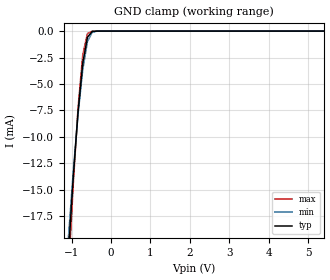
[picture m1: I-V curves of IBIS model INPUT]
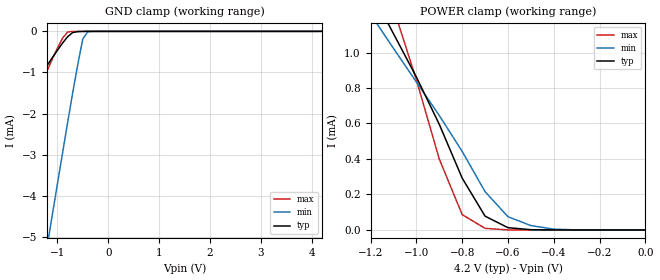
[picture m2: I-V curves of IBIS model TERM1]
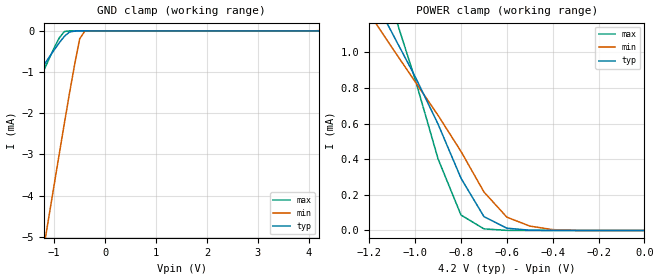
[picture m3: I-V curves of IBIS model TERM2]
|   PERICOM SEMICONDUCTOR CORP
|   IBIS Model of PI3A223
|   Product Family: 3A
|   UQFN-10 (ZM) Package
[IBIS Ver] 3.2
[Comment char] |_char
[File Name] pi3a223_zm_42v.ibs
[File Rev] 1.0
[Source] File originated at Pericom Semiconductor Corp.
[Date] 08/04/17
[Disclaimer] (C) Copyright PERICOM Semiconductor Corporation
   All rights reserved
  Pericom Semiconductor Corporation hereby grants the user of
  this IBIS model a non-exclusive, nontransferable license to
  use this IBIS model under the following terms.
  This IBIS model is provided on an "AS IS" basis and Pericom
  makes absolutely no warranty with respect to the information
  contained herein. PERICOM DISCLAIMS AND CUSTOMER WAIVES ALL
  WARRANTIES, EXPRESSED OR IMPLIED, INCLUDING WARRANTIES OF
  MERCHANTABILITY OR FITNESS FOR A PARTICULAR PURPOSE. The
  entire risk as to quality and performance is with the customer.
  Accordingly, in no event shall the company be liable for any
  damages, whether in contract or tort, including any lost
  profits or other incidental, consequential, exemplary, or
  punitive damages arising out of the use or application of the
  IBIS model provided in this package. Further, Pericom reserves
  the right to make changes without notice to any product herein
  to improve reliability, function, or design. Pericom does not
  convey any license under patent rights or any other intellectual
  property rights, including those of third parties.
  The user is granted this license only to use the IBIS model
  and is not granted rights to sell, load, rent, lease or license
  the IBIS model in whole or in part, or in modified form to anyone
  other than user. User may modify the IBIS model to suit its specific
  application but rights to derivative works and such modifications
  shall belong to Pericom.
  Pericom is not obligated to provide maintenance or support
  for the licensed IBIS model.
  Contact Pericom at ATTN: APPLICATION ENGINEERING / IBIS MODELS
  2380 Bering Drive, San Jose, CA 95131
[Component] PI3A223
[Manufacturer] Pericom Semiconductor Corp.
[Package]
| variable   typ   min   max
R_pkg   0.10120ohm   0.09060ohm   0.11180ohm
L_pkg   1.24800nH   1.01600nH   1.48000nH
C_pkg   0.22300pF   0.20300pF   0.24400pF
[Pin] signal_name   model_name   R_pin   L_pin   C_pin
1   VDD   POWER   0.10120   1.24800nH   0.22300pF
2   NO1   TERM1   0.10120   1.24800nH   0.22300pF
3   COM1   TERM2   0.11180   1.48000nH   0.24400pF
4   IN1   INPUT   0.09060   1.01600nH   0.20200pF
5   NC1   TERM1   0.11180   1.48000nH   0.24400pF
6   GND   GND   0.10120   1.24800nH   0.22300pF
7   NC2   TERM1   0.10120   1.24800nH   0.22300pF
8   IN2   INPUT   0.11180   1.48000nH   0.24400pF
9   COM2   TERM2   0.09060   1.01600nH   0.20200pF
10   NO2   TERM1   0.11180   1.48000nH   0.24400pF
[Series Switch Groups]
On 1 /
Off 2 /
[Series Pin Mapping]   pin_2   model_name  function_table_group
5   3   SWITCH1   1
2   3   SWITCH1   2
7   9   SWITCH1   1
10   9   SWITCH1   2
|   Model SWITCH1
[Model] SWITCH1
Model_type Series_switch
| variable   typ   min   max
C_comp   67.00pF   66.50pF   67.50pF
[Voltage Range]   4.2000V   3.7800V   4.6200V
[GND Clamp Reference]   0.0000V   0.0000V   0.0000V
[POWER Clamp Reference]   4.2000V   3.7800V   4.6200V
[Temperature Range]   25   85   -40
[On]
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[OFF]
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| Models and submodels in the file (4): INPUT (Input), SWITCH1 (Series_switch), TERM1 (Terminator), TERM2 (Terminator)
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|   Model INPUT
[Model] INPUT
Model_type Input
Vinl = 420mV
Vinh = 2.94V
| variable   typ   min   max
C_comp   0.950pF   0.940pF   0.960pF
[Voltage Range]   4.2000V   3.7800V   4.6200V
[GND Clamp Reference]   0.0000V   0.0000V   0.0000V
[POWER Clamp Reference]   4.2000V   3.7800V   4.6200V
[Temperature Range]   25   85   -40
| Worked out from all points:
|   GND clamp passes 1 mA (typ) near -0.62 V on its own axis
[GND Clamp]
| Voltage   I(typ)   I(min)   I(max)
-4.2V     -233.5mA   -213.1mA   -261.7mA
-1.08V    -20.87mA   -19.38mA   -22.91mA
-960mV    -13.8mA    -13.29mA   -14.48mA
-840mV    -7.703mA   -7.939mA   -7.326mA
-720mV    -3.053mA   -3.654mA   -2.254mA
-600mV    -576.6uA   -991.2uA   -224.1uA
-480mV    -38.17uA   -117.3uA   -5.86uA
-240mV    -22.46nA   -288.9nA   -320.8pA
8.4V      1.541nA    46.91nA    172.2pA
[POWER Clamp]   |Note: Vtable = Vcc - Voutput
| Voltage   I(typ)   I(min)   I(max)
-4.2V     0A         0A         0A
0V        0A         0A         0A
|   Model TERM1
[Model] TERM1
Model_type Terminator
| variable   typ   min   max
C_comp   26.00pF   25.80pF   26.20pF
[Voltage Range]   4.2000V   3.7800V   4.6200V
[GND Clamp Reference]   0.0000V   0.0000V   0.0000V
[POWER Clamp Reference]   4.2000V   3.7800V   4.6200V
[Temperature Range]   25   85   -40
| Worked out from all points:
|   GND clamp passes 1 mA (typ) near -1.29 V on its own axis
|   POWER clamp passes 1 mA (typ) near -1.06 V on its own axis
[GND Clamp]
| Voltage   I(typ)   I(min)   I(max)
-4.2V     -6.641mA   -27.99mA   -9.651mA
-3.3V     -4.881mA   -21.15mA   -7.019mA
-2.6V     -3.516mA   -15.83mA   -4.977mA
-2.5V     -3.322mA   -15.07mA   -4.686mA
-1.2V     -826.1uA   -5.218mA   -950.2uA
-1.1V     -641.5uA   -4.465mA   -675.9uA
-900mV    -288uA     -2.968mA   -169.2uA
-800mV    -132.1uA   -2.227mA   -15.8uA
-700mV    -28.51uA   -1.5mA     -151.1nA
-500mV    -1.252uA   -181.6uA   -2.028nA
-400mV    -28.38nA   -7.774uA   -1.598nA
4.2V      465.6pA    7.186uA    354.8pA
[POWER Clamp]   |Note: Vtable = Vcc - Voutput
| Voltage   I(typ)   I(min)   I(max)
-4.2V     10.64mA    9.052mA    14.23mA
-1.2V     1.351mA    1.216mA    1.609mA
-1.1V     1.106mA    1.024mA    1.25mA
-1V       862.1uA    834uA      846.5uA
-900mV    595.5uA    645.2uA    400.1uA
-800mV    292.3uA    442.7uA    86.46uA
-700mV    77.69uA    215.7uA    9.045uA
-600mV    12.83uA    74.63uA    509.8nA
-500mV    1.577uA    24.68uA    16.17nA
-400mV    61.81nA    4.683uA    1.355nA
0V        458.3pA    744pA      481.7pA
|   Model TERM2
[Model] TERM2
Model_type Terminator
| variable   typ   min   max
C_comp   41.0pF   40.7pF   41.3pF
[Voltage Range]   4.2000V   3.7800V   4.6200V
[GND Clamp Reference]   0.0000V   0.0000V   0.0000V
[POWER Clamp Reference]   4.2000V   3.7800V   4.6200V
[Temperature Range]   25   85   -40
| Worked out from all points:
|   GND clamp passes 1 mA (typ) near -1.29 V on its own axis
|   POWER clamp passes 1 mA (typ) near -1.06 V on its own axis
[GND Clamp]
| Voltage   I(typ)   I(min)   I(max)
-4.2V     -6.642mA   -28.02mA   -9.653mA
-3.3V     -4.882mA   -21.17mA   -7.02mA
-2.6V     -3.517mA   -15.85mA   -4.978mA
-2.5V     -3.322mA   -15.09mA   -4.687mA
-1.2V     -826.4uA   -5.231mA   -950.6uA
-1.1V     -641.8uA   -4.478mA   -676.2uA
-900mV    -288.2uA   -2.98mA    -169.3uA
-800mV    -132.2uA   -2.24mA    -15.8uA
-700mV    -28.52uA   -1.513mA   -166.8nA
-500mV    -1.253uA   -192.5uA   -2.028nA
-400mV    -28.39nA   -7.92uA    -1.595nA
4.2V      755.6pA    7.188uA    645.6pA
[POWER Clamp]   |Note: Vtable = Vcc - Voutput
| Voltage   I(typ)   I(min)   I(max)
-4.2V     10.65mA    9.056mA    14.24mA
-1.2V     1.352mA    1.217mA    1.611mA
-1.1V     1.107mA    1.025mA    1.252mA
-1V       863.1uA    834.7uA    848.3uA
-900mV    596.6uA    646uA      401.2uA
-800mV    292.9uA    443.5uA    86.6uA
-700mV    77.83uA    216.2uA    9.046uA
-600mV    12.83uA    74.78uA    509.9nA
-500mV    1.577uA    24.7uA     16.14nA
-400mV    61.81nA    4.684uA    1.449nA
0V        748.3pA    766.9pA    769.3pA
